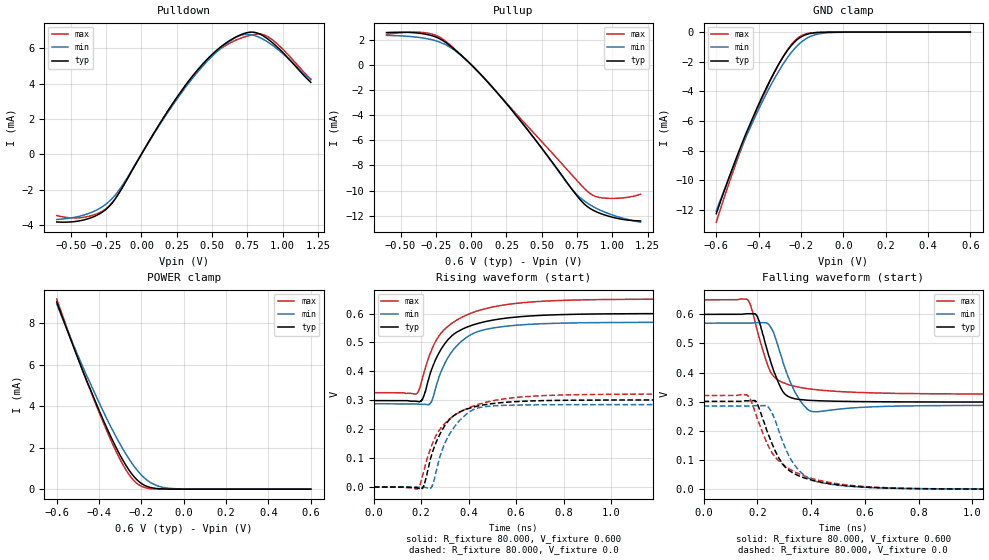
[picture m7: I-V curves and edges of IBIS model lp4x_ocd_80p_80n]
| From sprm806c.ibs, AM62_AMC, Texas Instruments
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|   Model lp4x_ocd_80p_80n
[Model] lp4x_ocd_80p_80n
Model_type I/O
Polarity   Non-Inverting
Enable   Active-High
Vinl =  0.0V
Vinh =  0.900V
Vmeas =  0.600V
C_comp   2.488pF   2.282pF   2.735pF
[Model Spec]
Vinh   0.900V   0.900V   0.900V
Vinl   0.0V   0.0V   0.0V
Vmeas   0.600V   NA   NA
[Temperature Range]   25.000   0.125k   -40.000
[Voltage Range]   0.600V   0.570V   0.650V
[Pullup Reference]   0.600V   0.570V   0.650V
[Pulldown Reference]   0.0V   0.0V   0.0V
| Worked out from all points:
|   slope of the pulldown table from 0 to 0.09 V, typ, clamps not added: 74 ohm
|   slope of the pullup table from 0 to 0.09 V, typ, clamps not added: 86.1 ohm
|   GND clamp passes 1 mA (typ) near -0.25 V on its own axis
|   POWER clamp passes 1 mA (typ) near -0.26 V on its own axis
|   rising waveform, R_fixture 80.000, V_fixture 0.600: 20-80 % time 132ps typ, 122ps min, 156ps max; typ from 0.299 V to 0.6 V
|   rising waveform, R_fixture 80.000, V_fixture 0.0: 20-80 % time 99.6ps typ, 95.8ps min, 145ps max; typ from 0 V to 0.301 V
|   falling waveform, R_fixture 80.000, V_fixture 0.600: 20-80 % time 63.4ps typ, 65.1ps min, 68.5ps max; typ from 0.6 V to 0.299 V
|   falling waveform, R_fixture 80.000, V_fixture 0.0: 20-80 % time 105ps typ, 93.5ps min, 134ps max; typ from 0.301 V to 0 V
[Pulldown]
|Voltage   I(typ)   I(min)   I(max)
-600mV    -3.84mA    -3.699mA   -3.476mA
-392mV    -3.691mA   -3.408mA   -3.551mA
-221mV    -2.888mA   -2.618mA   -2.88mA
-126mV    -1.762mA   -1.654mA   -1.752mA
120mV     1.608mA    1.553mA    1.601mA
328mV     4.08mA     3.962mA    4.066mA
499mV     5.646mA    5.542mA    5.589mA
669mV     6.648mA    6.625mA    6.469mA
783mV     6.925mA    6.768mA    6.766mA
878mV     6.633mA    6.446mA    6.738mA
992mV     5.848mA    5.771mA    6.028mA
1.2V      4.074mA    4.222mA    4.268mA
[Pullup]
|Voltage   I(typ)   I(min)   I(max)
-600mV    2.551mA    2.325mA    2.405mA
-297mV    2.36mA     2.029mA    2.483mA
-221mV    2.046mA    1.782mA    2.169mA
-107mV    1.101mA    1.049mA    1.141mA
44.21mV   -500.6uA   -496.7uA   -510.5uA
215mV     -2.634mA   -2.615mA   -2.609mA
461mV     -6.059mA   -6.075mA   -5.643mA
707mV     -9.795mA   -9.802mA   -8.683mA
840mV     -11.41mA   -11.12mA   -10.22mA
897mV     -11.74mA   -11.47mA   -10.52mA
992mV     -12.1mA    -11.91mA   -10.62mA
1.2V      -12.42mA   -12.52mA   -10.3mA
[GND_clamp]
|Voltage   I(typ)   I(min)   I(max)
-600mV    -12.26mA   -12.07mA   -12.83mA
-535mV    -9.631mA   -9.657mA   -9.998mA
-483mV    -7.674mA   -7.84mA    -7.926mA
-457mV    -6.749mA   -6.974mA   -6.957mA
-378mV    -4.198mA   -4.571mA   -4.306mA
-326mV    -2.706mA   -3.156mA   -2.747mA
-287mV    -1.735mA   -2.22mA    -1.722mA
-248mV    -949.7uA   -1.424mA   -887.8uA
-209mV    -414uA     -806.5uA   -336.6uA
-157mV    -95.45uA   -302uA     -61.63uA
-78.26mV  -9.109uA   -53.02uA   -8.174uA
600mV     0A         0A         0A
[POWER_clamp]
|Voltage   I(typ)   I(min)   I(max)
-600mV    9.037mA    8.928mA    9.175mA
-457mV    5.197mA    5.441mA    5.165mA
-352mV    2.698mA    3.164mA    2.544mA
-313mV    1.878mA    2.4mA      1.683mA
-274mV    1.164mA    1.707mA    946.7uA
-248mV    770.4uA    1.297mA    560.1uA
-222mV    461.7uA    938.4uA    283.8uA
-196mV    245.9uA    638.8uA    120.5uA
-157mV    79.31uA    316.3uA    23.58uA
-117mV    22.66uA    136.3uA    6.081uA
-78.26mV  6.702uA    54.45uA    1.892uA
600mV     0A         0A         0A
[Ramp]
| variable   typ   min   max
dV/dt_r   0.181/99.553p   0.171/95.850p   0.193/0.145n
dV/dt_f   0.181/63.248p   0.170/65.005p   0.195/68.519p
R_load = 80.000
[Rising Waveform]
R_fixture= 80.000
V_fixture= 0.600
V_fixture_min= 0.570
V_fixture_max= 0.650
|time   V(typ)   V(min)   V(max)
0s        298.9mV    287.8mV    326.3mV
183ps     296.1mV    287.1mV    324.2mV
205ps     302.4mV    286.3mV    377mV
235ps     385mV      286.2mV    457.2mV
298ps     494.2mV    426.6mV    545mV
363ps     541.8mV    499.2mV    583.8mV
436ps     565mV      537mV      608.7mV
579ps     586.1mV    558mV      633.1mV
1.023ns   599.1mV    569mV      648.8mV
3ns       600mV      569.7mV    650mV
[Rising Waveform]
R_fixture= 80.000
V_fixture= 0.0
V_fixture_min= 0.0
V_fixture_max= 0.0
|time   V(typ)   V(min)   V(max)
0s        107.9uV    560.3uV    101uV
184ps     -3.062mV   -291.7uV   -6.481mV
211ps     3.251mV    -852.1uV   55.69mV
239ps     98.01mV    -4.712mV   133.7mV
250ps     127.3mV    11.02mV    156.5mV
297ps     209.1mV    147.5mV    217.9mV
364ps     260.4mV    232.5mV    259.8mV
430ps     278.7mV    271.3mV    283.2mV
554ps     293mV      282.6mV    305.5mV
3ns       301.3mV    285mV      321.6mV
[Falling Waveform]
R_fixture= 80.000
V_fixture= 0.600
V_fixture_min= 0.570
V_fixture_max= 0.650
|time   V(typ)   V(min)   V(max)
0s        600mV      569.7mV    650mV
164ps     602.1mV    569.7mV    650.5mV
200ps     593.4mV    571.4mV    544.6mV
239ps     469.3mV    568.5mV    423.6mV
261ps     405.5mV    536.4mV    386.6mV
302ps     326.8mV    418.3mV    363.2mV
359ps     307.6mV    304.1mV    349.2mV
410ps     304.1mV    265.8mV    342.3mV
835ps     299.3mV    286.7mV    327.6mV
3ns       298.9mV    287.8mV    326.3mV
[Falling Waveform]
R_fixture= 80.000
V_fixture= 0.0
V_fixture_min= 0.0
V_fixture_max= 0.0
|time   V(typ)   V(min)   V(max)
0s        301.2mV    285mV      321.6mV
162ps     303.3mV    285mV      323.1mV
195ps     301.8mV    286.8mV    255.7mV
239ps     192.8mV    283.7mV    151.7mV
257ps     151.5mV    257.8mV    121.9mV
294ps     87.09mV    163.3mV    85.37mV
353ps     46.45mV    66.41mV    53.47mV
411ps     29.14mV    28.75mV    34.84mV
536ps     11.22mV    10.47mV    14.2mV
3ns       105.7uV    552.2uV    98.84uV
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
